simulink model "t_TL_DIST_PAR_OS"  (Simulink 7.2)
settings: Solver=ode3  SolverMode=SingleTasking  StartTime=0.0  StopTime=0.05  FixedStep=10e-6  MaxStep=1e-5  RelTol=1e-5  AbsTol=1e-5

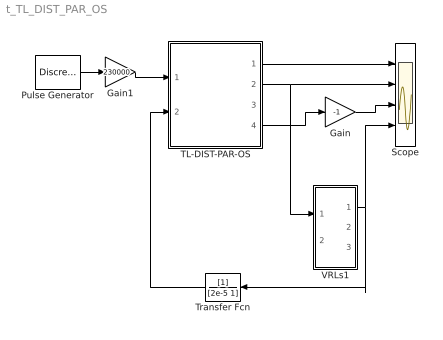
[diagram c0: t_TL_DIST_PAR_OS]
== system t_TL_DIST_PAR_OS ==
  Gain : Gain  Gain=-1  ParameterDataType=sfix(16)  ParameterScaling=2^0  OutDataType=sfix(16)  OutScaling=2^0
  Gain1 : Gain  Gain=230000  ParameterDataType=sfix(16)  ParameterScaling=2^0  OutDataType=sfix(16)  OutScaling=2^0
  Pulse Generator : DiscretePulseGenerator  PulseType=Time based  Period=0.02  PulseWidth=50
  Scope : Scope  NumInputPorts=4
  TL-DIST-PAR-OS : Subsystem  mask(1-Phase TL-DIST-PAR){L=1.3e-3, C=8.9e-9, R=0.05, TL=200, RS=50}
      mask prompts: L "L/km"; C "C/km"; R "R/km"; TL "Length[km]"
      mask help: 1 Phase frequency independent trans. Line based on the Bergerons model. Input Vector: u[0]=Input Voltage u[1]=Load Current Output Vector: y[0]=Input Voltage y[1]=Output Voltage y[2]=Input Current y[3]=Output Current PArameter Vector: p[0]= TL-Inductane L/km p[1]= TL-Capacitance C/km p[2]= TL-Resistance R/km p[3]= TL-Length [km] p[4]= TL-Input Resistance R
  Transfer Fcn : TransferFcn  Orientation=left  Denominator=[2e-5 1]
  VRLs1 : Subsystem  mask(VRLs_OS){R=380+380, L=1e-3, IL0=0, RLp=1e6}
      mask prompts: R "Output Resistance"; L "Output Inductance"; IL0 "Initial Inductor Current"; RLp "Ind. Parallel Res"
      mask help: Open source VRL_Series Input Vector: u[0]= Vs, Source Voltage u[1]= E, Load Voltage Output Vector: y[0]=IL, Load current y[1]=VL, Inductance Voltage y[2]=VR, Resistance Voltage Parameter Vector: p[0]=R p[1]=L p[2]=IL0
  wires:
  TL-DIST-PAR-OS/2(TL_V_OUT) -> VRLs1/1(v), Scope/2
  TL-DIST-PAR-OS/4(TL_I_OUT) -> Gain/1
  Pulse Generator/1 -> Gain1/1
  Gain1/1 -> TL-DIST-PAR-OS/1(V_In)
  Transfer Fcn/1 -> TL-DIST-PAR-OS/2(I_Load)
  VRLs1/1(iL) -> Scope/4, Transfer Fcn/1
  TL-DIST-PAR-OS/1(TL_V_IN) -> Scope/1
  Gain/1 -> Scope/3

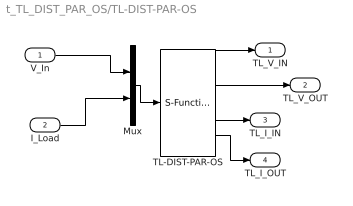
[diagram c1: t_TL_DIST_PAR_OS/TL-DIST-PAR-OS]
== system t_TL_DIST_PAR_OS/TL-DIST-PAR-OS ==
  V_In : Inport  OutDataType=sfix(16)  OutScaling=2^0
  I_Load : Inport  Port=2  OutDataType=sfix(16)  OutScaling=2^0
  Mux : Mux  Inputs=2
  TL-DIST-PAR-OS : S-Function  FunctionName=s_TL_DIST_PAR_OS  Parameters=[L C R TL RS ]  EnableBusSupport=off
  TL_V_IN : Outport  OutDataType=sfix(16)  OutScaling=2^0
  TL_V_OUT : Outport  Port=2  OutDataType=sfix(16)  OutScaling=2^0
  TL_I_IN : Outport  Port=3  OutDataType=sfix(16)  OutScaling=2^0
  TL_I_OUT : Outport  Port=4  OutDataType=sfix(16)  OutScaling=2^0
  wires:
  TL-DIST-PAR-OS/3 -> TL_I_IN/1
  TL-DIST-PAR-OS/2 -> TL_V_OUT/1
  TL-DIST-PAR-OS/1 -> TL_V_IN/1
  I_Load/1 -> Mux/2
  V_In/1 -> Mux/1
  Mux/1 -> TL-DIST-PAR-OS/1
  TL-DIST-PAR-OS/4 -> TL_I_OUT/1

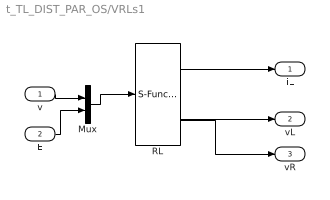
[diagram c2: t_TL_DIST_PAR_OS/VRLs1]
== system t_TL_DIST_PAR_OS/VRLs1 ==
  v : Inport
  E : Inport  Port=2
  Mux : Mux  Inputs=2
  RL : S-Function  FunctionName=s_VRLs_OS  Parameters=[R, L, IL0, RLp]  EnableBusSupport=off
  iL : Outport
  vL : Outport  Port=2
  vR : Outport  Port=3
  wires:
  Mux/1 -> RL/1
  E/1 -> Mux/2
  v/1 -> Mux/1
  RL/1 -> iL/1
  RL/2 -> vL/1
  RL/3 -> vR/1
